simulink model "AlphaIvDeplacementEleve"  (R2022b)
settings: Solver=VariableStepAuto  StartTime=0.0  StopTime=15  RelTol=1e-3
libraries: fl_lib x8, nesl_utility x5, ee_lib x1

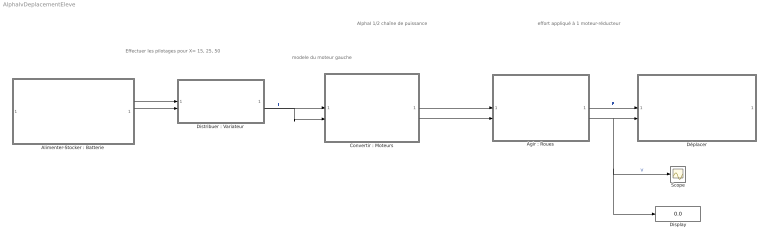
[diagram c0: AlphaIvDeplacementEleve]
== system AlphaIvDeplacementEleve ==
  note: Effectuer les pilotages pour X= 15, 25, 50
  note: modele du moteur gauche
  note: AlphaI 1/2 chaîne de puissance
  note: effort appliqué à 1 moteur-réducteur
  "Agir : Roues" : Subsystem  mask{R=0.044/2}
      mask prompts: R "Rayon de la roue (m)"
  "Alimenter-Stocker : Batterie" : Subsystem  mask{Uchar=8.36, Ucoup=5.92, Q=0.65, Irobot=0.3, N=2}
      mask prompts: Uchar "Tension fin charge (V)"; Ucoup "Tension de coupure (V)"; Q "Capacité (en  Ah)"; Irobot "Intensité en (A) robot à l'arrêt"; N "Nombre de chaine de puissance"
  "Convertir : Moteurs" : Subsystem  mask{I0=0.1, Umot=0, k=0, N0=0, Cmax=0}
      mask prompts: I0 "Courant à Vide (A)"; Umot "Tension Moteur (V)"; k "Rapport de transmisson"; N0 "Vitesse à vide(en RPM)"; Cmax "Couple rotor bloqué (Nm)"
  Display : Display
  "Distribuer : Variateur" : Subsystem  mask{v=0.0}
      mask prompts: v "Valeur X de pilotage par rapport à la commande motor(X,X,temps) du programme python"
  Déplacer : Subsystem  mask{masseProduit=0.4/2, Crr=0.047, pente=0}
      mask prompts: masseProduit "Masse du produit appliquée à une roue en kg"; Crr "Coefficient de résistance au roulement"; pente "pente en %"
  Scope : Scope
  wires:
  "Convertir : Moteurs"/2(w reducteur) -> "Agir : Roues"/2(wreducteur)
  "Convertir : Moteurs"/1(Couple reducteur) -> "Agir : Roues"/1(Creducteur)
  "Distribuer : Variateur"/2(Out2) -> "Convertir : Moteurs"/2(In2)  "I"
  "Distribuer : Variateur"/1(Out1) -> "Convertir : Moteurs"/1(In1)
  "Alimenter-Stocker : Batterie"/1(Out1) -> "Distribuer : Variateur"/1(In1)
  "Alimenter-Stocker : Batterie"/2(Out2) -> "Distribuer : Variateur"/2(In2)  "I"
  "Agir : Roues"/1(Froue) -> Déplacer/1(In2)  "F"
  "Agir : Roues"/2(V(m/s)) -> Display/1, Scope/1, Déplacer/2(In1)  "V"

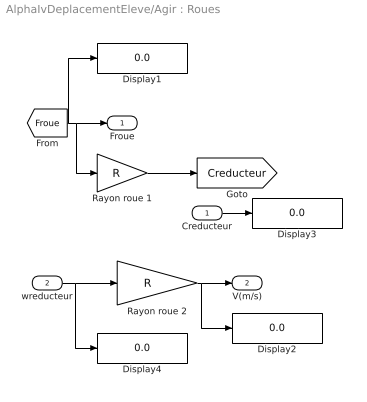
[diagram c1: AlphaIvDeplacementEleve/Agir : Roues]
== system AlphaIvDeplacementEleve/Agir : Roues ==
  Creducteur : Inport
  wreducteur : Inport  Port=2
  Display{1..4} (4 alike) : Display
  Rayon roue 1 : Gain  Gain=R
  Rayon roue 2 : Gain  Gain=R
  Froue : Outport  VectorParamsAs1DForOutWhenUnconnected=off
  V(m/s) : Outport  Port=2  VectorParamsAs1DForOutWhenUnconnected=off
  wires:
  wreducteur/1 -> Display4/1, Rayon roue 2/1
  Rayon roue 2/1 -> Display2/1, V(m/s)/1
  [Froue] -> Display1/1, Rayon roue 1/1, Froue/1
  Creducteur/1 -> Display3/1
  Rayon roue 1/1 -> [Creducteur]

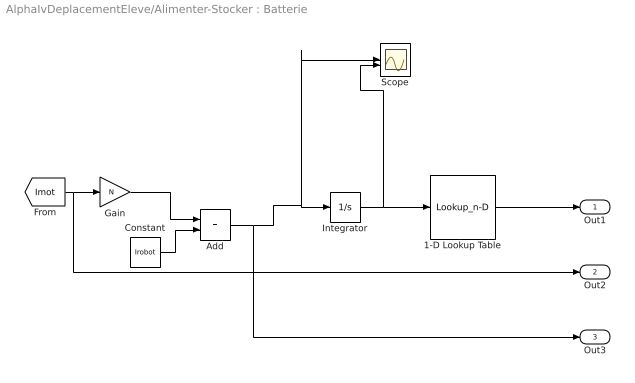
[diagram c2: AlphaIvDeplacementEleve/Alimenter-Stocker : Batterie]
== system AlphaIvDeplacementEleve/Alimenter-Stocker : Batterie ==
  1-D Lookup Table : Lookup_n-D  NumberOfTableDimensions=1  BreakpointsForDimension1=[0;Q*3600]  Table=[Uchar;Ucoup]  InternalRulePriority=Speed  RndMeth=Simplest
  Add : Sum
  Constant : Constant  Value=Irobot
  Gain : Gain  Gain=N
  Integrator : Integrator
  Scope : Scope  NumInputPorts=2
  Out1 : Outport  VectorParamsAs1DForOutWhenUnconnected=off
  Out2 : Outport  Port=2  VectorParamsAs1DForOutWhenUnconnected=off
  Out3 : Outport  Port=3  VectorParamsAs1DForOutWhenUnconnected=off
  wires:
  1-D Lookup Table/1 -> Out1/1
  Add/1 -> Out3/1, Scope/1, Integrator/1
  Integrator/1 -> Scope/2, 1-D Lookup Table/1
  [Imot] -> Out2/1, Gain/1
  Constant/1 -> Add/2
  Gain/1 -> Add/1

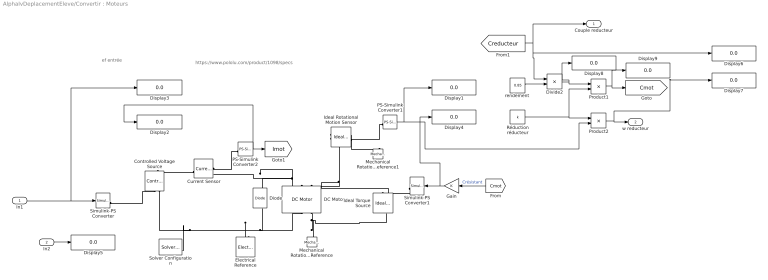
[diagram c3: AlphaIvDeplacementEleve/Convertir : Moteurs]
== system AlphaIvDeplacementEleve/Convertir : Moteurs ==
  note: ef entrée
  note: https://www.pololu.com/product/1098/specs
  In1 : Inport
  In2 : Inport  Port=2
  Controlled Voltage Source : fl_lib/Electrical/Electrical Sources/Controlled Voltage Source
  Current Sensor : fl_lib/Electrical/Electrical Sensors/Current Sensor
  DC Motor : ee_lib/Electromechanical/Brushed Motors/DC Motor  field_option=ee.enum.field_option.pm  Rf=100 Ohm  Lf=1 H  Laf=0.15 H  If0=0 A  parameterization=2  Ra=0.35 Ohm  La=5.61e-3 mH  emf_or_torque=1  Kv=0.1 V/(rad/s)  Ki=0.105 N*m/A  T_stall=(Cmax)/(30*0.85) N*m  w_max=N0/k rpm  w_rated=2000 rpm  P_rated=1000 W  V_rated=Umot V  lam_param=2  i_noload=I0 A  V_i_noload=Umot V  J=0.340 g*cm^2  lam=1e-8 N*m/(rad/s)  speed0=0 rpm  enable_fault_armature=simscape.enum.onoff.off  rev_faulted=1 / 3  G_faulted_armature=1e-5 S  fault_trigger_armature=ee.enum.faults.faultTrigger.temporal  t_fault_armature=1 s  max_permissible_current_armature=inf A  t_fail_on_current_armature=1 s  enable_fault_field=simscape.enum.onoff.off  G_faulted_field=1e-5 S  fault_trigger_field=ee.enum.faults.faultTrigger.temporal  t_fault_field=1 s  max_permissible_current_field=inf A  t_fail_on_current_field=1 s  fault_action=simscape.enum.assert.action.none  alpha=3.93e-3 1/K  Tmeas=25 degC  thermal_mass=100 J/K  initial_temperature=25 degC
  Diode : fl_lib/Electrical/Electrical Elements/Diode  Vf=0.6 V  Ron=0.3 Ohm  Goff=1e-8 1/Ohm  i_specify=off  i_priority=None  i=0 A  i_nominal_specify=off  i_nominal_unit=A  i_nominal_value=1  v_specify=off  v_priority=None  v=0 V  v_nominal_specify=off  v_nominal_unit=V  v_nominal_value=1
  Display{1..9} (9 alike) : Display
  Divide2 : Product  Inputs=*/
  Electrical Reference : fl_lib/Electrical/Electrical Elements/Electrical Reference
  Gain : Gain
  Ideal Rotational Motion Sensor : fl_lib/Mechanical/Mechanical Sensors/Ideal Rotational Motion Sensor  reference=foundation.enum.MeasurementReference.difference  acceleration_port=false  velocity_port=true  position_port=true  wrap_angle=false  offset=0 rad
  Ideal Torque Source : fl_lib/Mechanical/Mechanical Sources/Ideal Torque Source
  Mechanical Rotational Reference : fl_lib/Mechanical/Rotational Elements/Mechanical Rotational Reference
  Mechanical Rotational Reference1 : fl_lib/Mechanical/Rotational Elements/Mechanical Rotational Reference
  PS-Simulink Converter1 : nesl_utility/PS-Simulink Converter  PhysicalDomain=network_engine_domain  SubClassName=ps_output  LeftPortType=input  RightPortType=output  PseudoPeriodic=off  Frequencies=[]  VectorFormat=1-D array  Unit=rad/s  AffineConversion=off
  PS-Simulink Converter2 : nesl_utility/PS-Simulink Converter  PhysicalDomain=network_engine_domain  SubClassName=ps_output  LeftPortType=input  RightPortType=output  PseudoPeriodic=off  Frequencies=[]  VectorFormat=1-D array  Unit=1  AffineConversion=off
  Product1 : Product  RndMeth=Zero
  Product2 : Product  Inputs=**
  Réduction réducteur : Constant  Value=k
  Simulink-PS Converter : nesl_utility/Simulink-PS Converter  PhysicalDomain=network_engine_domain  SubClassName=ps_input  LeftPortType=input  RightPortType=output  PseudoPeriodic=off  Frequencies=[]  NoiseDistribution=none  NoiseParameters=[]  Unit=1  AffineConversion=off  FilteringAndDerivatives=provide  SimscapeFilterOrder=1  InputFilterTimeConstant=0.001  UdotUserProvided=0
  Simulink-PS Converter1 : nesl_utility/Simulink-PS Converter  PhysicalDomain=network_engine_domain  SubClassName=ps_input  LeftPortType=input  RightPortType=output  PseudoPeriodic=off  Frequencies=[]  NoiseDistribution=none  NoiseParameters=[]  Unit=N*m  AffineConversion=off  FilteringAndDerivatives=zero  SimscapeFilterOrder=1  InputFilterTimeConstant=.001  UdotUserProvided=0
  Solver Configuration : nesl_utility/Solver Configuration  PhysicalDomain=network_engine_domain  SubClassName=solver  LeftPortType=input  RightPortType=generic  Tones=[]  Harmonics=[]  SimulateNoise=off  Profile=off  UseLocalSampling=off  EnableSwitchedLinearOptims=on  FrequencyDomain=off  UseCCode=off  RelTol=0.001  AbsTol=1e-06  MinStep=1e-09  ToWorkspace=off  RevertToSquareIcSolve=off  NumHomotopyIterations=100  PhasorMode=off  PhasorModeNumHarmonics=1  ConsistencySolver=NEWTON_FTOL  IndexReductionMethod=DerivativeReplacement  DoDC=off  ResidualTolerance=1e-9  ConsistencyTolSource=GLOBAL  ConsistencyAbsTol=0.001  ConsistencyRelTol=0.001  ConsistencyTolFactor=0.001  UseLocalSolver=on  LocalSolverChoice=NE_BACKWARD_EULER_ADVANCER  ResolveIndetEquations=on  FunctionEvalNumThread=1  LocalSolverSampleTime=.001  DoFixedCost=on  MaxNonlinIter=3  MaxModeIter=2  ComputeImpulses=off  ImpulseIterations=2  LinearAlgebra=Sparse  LinearAlgebraNumThread=0  EquationFormulation=NE_TIME_EF  DelaysMemoryBudget=1024  AutomaticFiltering=on  FilteringTimeConstant=0.001  PartitionStorageMethod=AS_NEEDED  PartitionMemoryBudget=1024  PartitionMethod=FAST
  "rendement " : Constant  Value=0.85  VectorParams1D=off
  Couple reducteur : Outport  VectorParamsAs1DForOutWhenUnconnected=off
  w reducteur : Outport  Port=2  VectorParamsAs1DForOutWhenUnconnected=off
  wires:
  [Cmot] -> Gain/1  "Crésistant"
  In2/1 -> Display5/1
  Gain/1 -> Simulink-PS Converter1/1, Display4/1
  In1/1 -> Simulink-PS Converter/1, Display3/1
  PS-Simulink Converter2/1 -> Display2/1, [Imot]
  Product1/1 -> Display9/1, [Cmot]
  Divide2/1 -> Display8/1, Product1/1
  "rendement "/1 -> Divide2/2
  PS-Simulink Converter1/1 -> Product2/2, Display1/1
  Réduction réducteur/1 -> Product2/1, Product1/2
  Product2/1 -> Display7/1, w reducteur/1
  [Creducteur] -> Divide2/1, Display6/1, Couple reducteur/1
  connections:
  Ideal Rotational Motion Sensor/RConn1 -- Mechanical Rotational Reference1/LConn1
  PS-Simulink Converter1/LConn1 -- Ideal Rotational Motion Sensor/RConn2
  DC Motor/LConn1 -- Diode/RConn1 -- Current Sensor/RConn2
  DC Motor/RConn2 -- Ideal Torque Source/LConn1 -- Mechanical Rotational Reference/LConn1
  Electrical Reference/LConn1 -- Diode/LConn1 -- DC Motor/RConn1 -- Solver Configuration/RConn1 -- Controlled Voltage Source/RConn2
  Ideal Rotational Motion Sensor/LConn1 -- Ideal Torque Source/RConn2 -- DC Motor/LConn2
  Simulink-PS Converter/RConn1 -- Controlled Voltage Source/RConn1
  Current Sensor/LConn1 -- Controlled Voltage Source/LConn1
  PS-Simulink Converter2/LConn1 -- Current Sensor/RConn1
  Simulink-PS Converter1/RConn1 -- Ideal Torque Source/RConn1

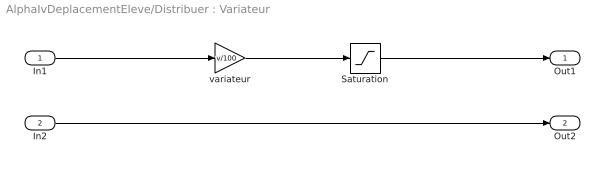
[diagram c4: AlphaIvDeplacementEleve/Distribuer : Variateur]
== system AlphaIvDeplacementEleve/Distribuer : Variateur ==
  In1 : Inport
  In2 : Inport  Port=2
  Saturation : Saturate  UpperLimit=4
  variateur : Gain  Gain=v/100
  Out1 : Outport
  Out2 : Outport  Port=2
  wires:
  In1/1 -> variateur/1
  variateur/1 -> Saturation/1
  In2/1 -> Out2/1
  Saturation/1 -> Out1/1

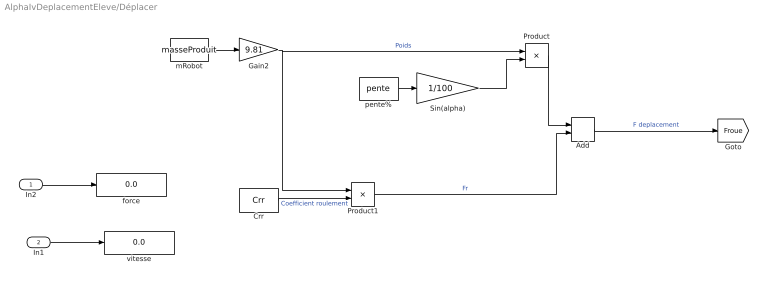
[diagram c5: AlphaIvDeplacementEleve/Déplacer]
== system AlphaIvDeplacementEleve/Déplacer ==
  In2 : Inport
  In1 : Inport  Port=2
  Add : Sum
  Crr : Constant  Value=Crr
  Gain2 : Gain  Gain=9.81
  Product : Product  RndMeth=Zero
  Product1 : Product  RndMeth=Zero
  Sin(alpha) : Gain  Gain=1/100
  force : Display
  mRobot : Constant  Value=masseProduit
  pente% : Constant  Value=pente
  vitesse : Display
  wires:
  Gain2/1 -> Product/1, Product1/1  "Poids"
  Product/1 -> Add/1
  pente%/1 -> Sin(alpha)/1
  Crr/1 -> Product1/2  "Coefficient roulement"
  mRobot/1 -> Gain2/1
  In1/1 -> vitesse/1
  In2/1 -> force/1
  Sin(alpha)/1 -> Product/2
  Product1/1 -> Add/2  "Fr"
  Add/1 -> [Froue]  "F deplacement"
